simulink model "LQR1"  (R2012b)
settings: Solver=ode45  StartTime=0.0  StopTime=10.0  RelTol=1e-3
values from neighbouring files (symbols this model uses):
  A = [0 1 0 0 0 0    [beobachter_1.m]    (also in beobachter_2.m; beobachter_22.m; kalman_1.m = my_sys.a; kalman_10.m = my_sys.a)
  B = [0 1 0 0 0 0]'    [beobachter_1.m]    (also in beobachter_2.m; beobachter_22.m; kalman_1.m = my_sys.b; kalman_10.m = my_sys.b)
  C = [0 0 0 0 1 0]    [beobachter_1.m]    (also in beobachter_2.m; beobachter_22.m; kalman_1.m = my_sys.c; kalman_10.m = my_sys.c)
  K = Kn(1:n)    [beobachter_2.m]    (also in beobachter_22.m; LQG_1.m = lqry(sys,10,1); LQR_1.m = Kn(1:6),      ki = -Kn(7),; pol_4.m)
  ki = -Kn(n+1)    [beobachter_2.m]    (also in beobachter_22.m; kalman_12.m = -Kn(3); kalman_13.m = -Kn(4); kalman_d1.m = -Kn(4))
  x0 = [30,-20,0,0,0,0]    [beobachter_1.m]    (also in beobachter_2.m = [0,0,0,0,0.3,0]; beobachter_22.m = [0.1,0,0.1,0,0.3,0]; kalman_13.m = zeros(1,3); kalman_d1.m = zeros(1,3))

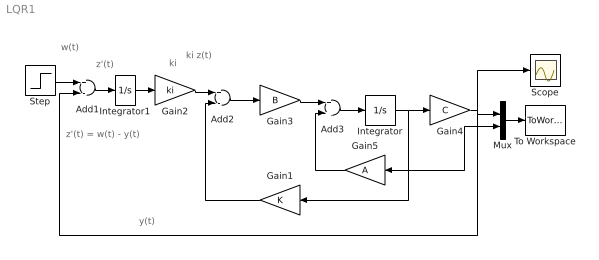
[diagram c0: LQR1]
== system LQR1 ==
  note: ki z(t)
  note: z'(t)
  note: ki
  note: z'(t) = w(t) - y(t)
  note: y(t)
  note: w(t)
  Add1 : Sum  Inputs=+-
  Add2 : Sum  Inputs=+-
  Add3 : Sum
  Gain1 : Gain  Gain=K  Multiplication=Matrix(K*u)
  Gain2 : Gain  Gain=ki
  Gain3 : Gain  Gain=B  Multiplication=Matrix(K*u)
  Gain4 : Gain  Gain=C  Multiplication=Matrix(K*u)
  Gain5 : Gain  Gain=A  Multiplication=Matrix(K*u)
  Integrator : Integrator  InitialCondition=x0
  Integrator1 : Integrator
  Mux : Mux  Inputs=2
  Scope : Scope
  Step : Step  Time=0  SampleTime=0
  To Workspace : ToWorkspace  VariableName=yx  SampleTime=-1  SaveFormat=Structure With Time
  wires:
  Step/1 -> Add1/1
  Add1/1 -> Integrator1/1
  Add2/1 -> Gain3/1
  Gain2/1 -> Add2/1
  Gain1/1 -> Add2/2
  Mux/1 -> To Workspace/1
  Gain3/1 -> Add3/1
  Add3/1 -> Integrator/1
  Gain4/1 -> Scope/1, Add1/2, Mux/1
  Gain5/1 -> Add3/2
  Integrator/1 -> Gain1/1, Mux/2, Gain5/1, Gain4/1
  Integrator1/1 -> Gain2/1
